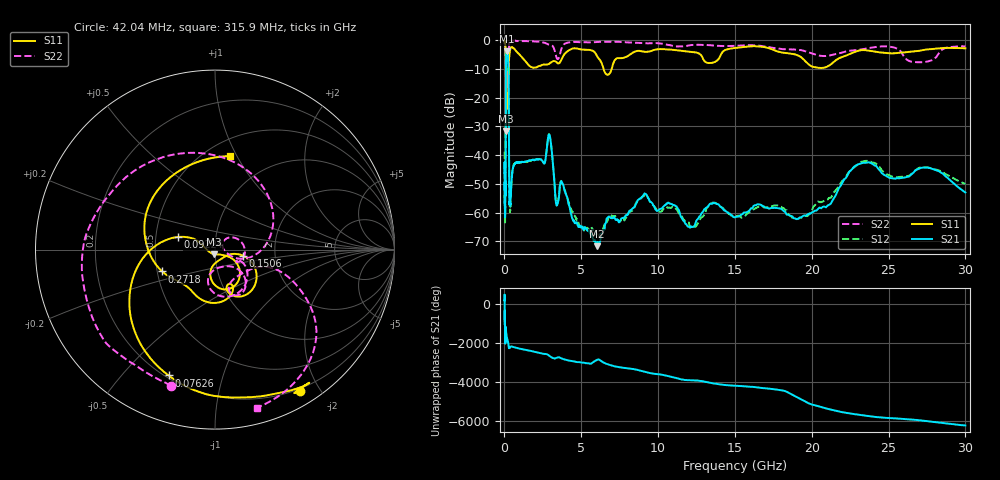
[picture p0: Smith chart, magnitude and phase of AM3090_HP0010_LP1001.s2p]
! Date/Time: Thu, Feb 28, 2019 1:55 PM
! Network Analyzer: Agilent Technologies E8364B Rev: A.07.50.67
! Sweep from 0.010 to 30.000 GHz, 1601 Points, Sweep Type: LOG
! Power Supply: 5.023 V, 0.002 A
# Hz S DB R 50
!freq MagS11 AngS11 MagS21 AngS21 MagS12 AngS12 MagS22 AngS22
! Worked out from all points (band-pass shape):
!   1601 points, 10 MHz to 30 GHz, reference 50 ohm
!   highest |S21| = -3.84 dB at 151.4 MHz (marker M1); lowest = -71.7 dB at 6.019 GHz (marker M2)
!   |S21| within 3 dB of the highest: 101.5 MHz to 248.8 MHz (147.3 MHz wide, 84.1 % of centre)
!   lowest |S11| = -31.8 dB at 99.92 MHz (marker M3), VSWR 1.05, Z = 49.3 - j2.47 ohm
!   |S11| at or under -10 dB: 90.64 MHz to 271.5 MHz (180.9 MHz wide, 99.9 % of centre); 6.45 GHz to 6.981 GHz (530.3 MHz wide, 7.9 % of centre)
!   |S22| runs from -27.0 to -0.1 dB; largest |S21 - S12| = 0.016
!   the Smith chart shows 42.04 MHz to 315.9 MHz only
!   S11 on the Smith chart (normalised r, x): 42.04 MHz: 0.17, -1.76; 76.26 MHz: 0.21, -0.68; 92.24 MHz: 0.65, +0.10; 150.6 MHz: 1.37, -0.10; 271.8 MHz: 0.53, -0.14; 315.9 MHz: 0.65, +0.94
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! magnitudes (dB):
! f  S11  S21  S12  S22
! 10 MHz  -0.3  -46.3  -38.8  -0.7
! 38.04 MHz  -0.5  -61.3  -61.3  -1.6
! 42.04 MHz  -0.7  -60.5  -60.3  -1.9
! 76.26 MHz  -2.5  -45.1  -44.5  -4.6
! 92.24 MHz  -13.2  -14.1  -14.0  -12.3
! 99.92 MHz  -31.8  -7.4  -7.4  -26.2
! 116.1 MHz  -12.9  -4.9  -4.9  -17.1
! 144.7 MHz  -21.4  -3.9  -3.9  -17.1
! 150.6 MHz  -15.9  -3.8  -3.8  -15.7
! 151.4 MHz  -15.4  -3.8  -3.8  -15.5
! 271.8 MHz  -9.9  -15.1  -15.0  -8.6
! 315.9 MHz  -5.5  -55.9  -55.3  -0.8
! 550.5 MHz  -2.7  -44.6  -44.4  -0.2
! 2.084 GHz  -9.5  -41.5  -41.4  -0.5
! 2.928 GHz  -8.2  -33.0  -33.0  -1.6
! 3.402 GHz  -7.7  -57.6  -56.9  -6.3
! 3.76 GHz  -6.1  -49.6  -49.9  -2.3
! 6.019 GHz  -5.5  -71.7  -67.6  -0.7
! 7.926 GHz  -5.8  -60.8  -61.7  -0.8
! 19.22 GHz  -5.6  -61.7  -61.9  -3.4
! 23.36 GHz  -3.5  -42.7  -42.2  -3.1
! 30 GHz  -2.9  -53.0  -50.0  -2.2
